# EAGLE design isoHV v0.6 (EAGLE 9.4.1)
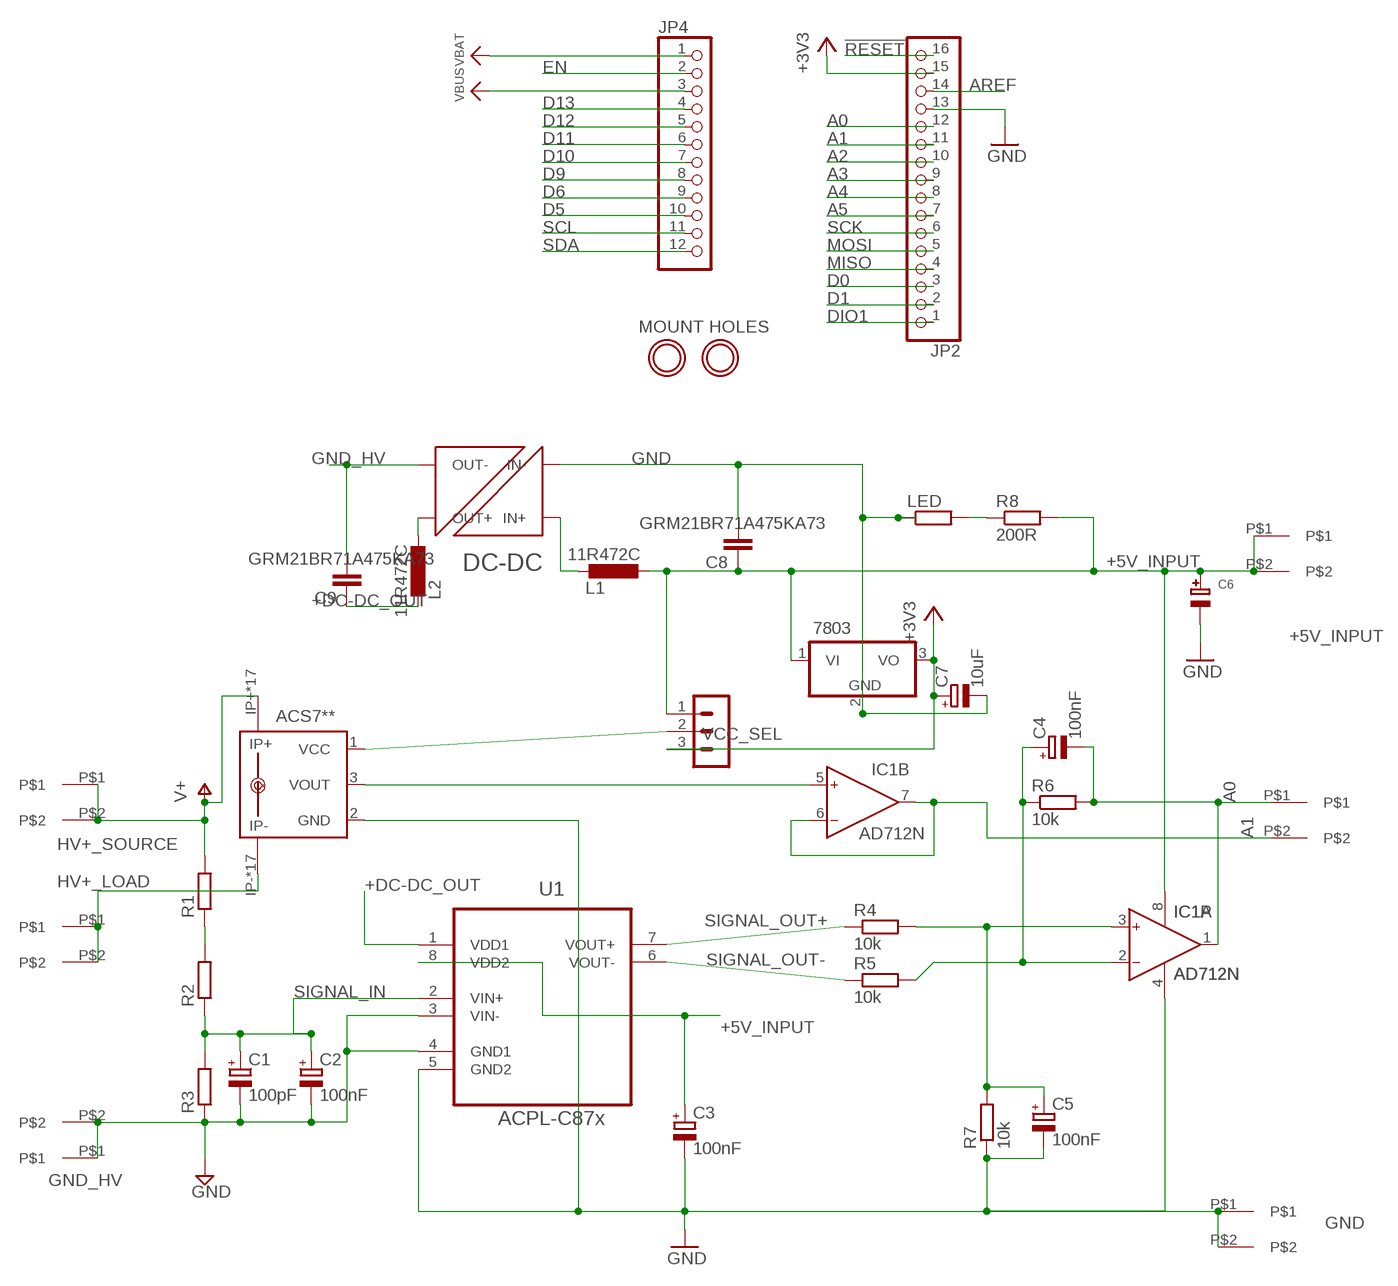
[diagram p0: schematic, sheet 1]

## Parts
7803  7805TV  [TO220V]
ACS7**  ACS758KCB-150B-PFF-T  [CB-PFF]
C1  100pF  CPOL-EUB45181A  [B45181A]
C2  100nF  CPOL-EUB45181A  [B45181A]
C3  100nF  CPOL-EUB45181A  [B45181A]
C4  100nF  CPOL-EUB45181A  [B45181A]
C5  100nF  CPOL-EUB45181A  [B45181A]
C6  CAP_ELECTROLYTICPTH_3.5MMGRID_10MMDIA  [CELEC_3.5MM_10MM]
C7  10uF  CPOL-EUB45181A  [B45181A]
C8  GRM21BR71A475KA73  C-EU025-050X050  [C025-050X050]
C9  GRM21BR71A475KA73  C-EU025-050X050  [C025-050X050]
IC1  AD712N  [DIL08]
JP2  HEADER-1X16ROUND  [1X16_ROUND]
JP4  HEADER-1X12  [1X12_ROUND]
L1  11R472C  L-EU0204V  [0204V]
L2  11R472C  L-EU0204V  [0204V]
LED  R-EU_0204/2V  [0204V]
R1  R-EU_0411/15  [0411/15]
R2  R-EU_0411/15  [0411/15]
R3  R-EU_0411/15  [0411/15]
R4  10k  R-EU_0204/7  [0204/7]
R5  10k  R-EU_0204/7  [0204/7]
R6  10k  R-EU_0204/7  [0204/7]
R7  10k  R-EU_0204/7  [0204/7]
R8  200R  R-EU_0204/2V  [0204V]
U1  ACPL-C87x  ACPL-C79B-000E  [SOIC127P1150X330-8N]
U$1  7.62MM_TERMINAL_BLOCK  [7.62MM]
U$2  7.62MM_TERMINAL_BLOCK  [7.62MM]
U$3  7.62MM_TERMINAL_BLOCK  [7.62MM]
U$4  7.62MM_TERMINAL_BLOCK  [7.62MM]
U$5  7.62MM_TERMINAL_BLOCK  [7.62MM]
U$6  7.62MM_TERMINAL_BLOCK  [7.62MM]
U$7  NXF1  [NXF1]
U$12  MOUNTINGHOLE2.5  [MOUNTINGHOLE_2.5_PLATED]
U$13  MOUNTINGHOLE2.5  [MOUNTINGHOLE_2.5_PLATED]
VCC_SEL  MA03-1  [MA03-1]

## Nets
!RESET: JP2.16
+3V3: 7803.3(VO) C7.+ JP2.15 VCC_SEL.3
+5V_INPUT: 7803.1(VI) C3.+ C6.+ C8.1 IC1.8(P:V+) L1.2 R8.2 U1.8(VDD2) U$3.P$1 U$3.P$2 VCC_SEL.1
+DC-DC_OUT: C9.1 L2.1 U1.1(VDD1)
A0: C4.- IC1.1(A:OUT) JP2.12 R6.2 U$5.P$1
A1: IC1.6(B:IN-) IC1.7(B:OUT) JP2.11 U$5.P$2
A2: JP2.10
A3: JP2.9
A4: JP2.8
A5: JP2.7
AREF: JP2.14
D0: JP2.3
D1: JP2.2
D5: JP4.10
D6: JP4.9
D9: JP4.8
D10: JP4.7
D11: JP4.6
D12: JP4.5
D13: JP4.4
DIO1: JP2.1
EN: JP4.2
GND: 7803.2(GND) ACS7**.2(GND) C3.- C5.- C6.- C7.- C8.2 IC1.4(P:V-) JP2.13 LED.1 R7.1 U1.5(GND2) U$4.P$1 U$4.P$2 U$7.P$1(IN-)
GND_HV: C1.- C2.- C9.2 R3.1 U1.3(VIN-) U1.4(GND1) U$2.P$1 U$2.P$2 U$7.P$7(OUT-) ; supply symbol labelled GND
HV+_LOAD: ACS7**.IP- ACS7**.IP-@2(IP-) ACS7**.IP-@3(IP-) ACS7**.IP-@4(IP-) ACS7**.IP-@5(IP-) ACS7**.IP-@6(IP-) ACS7**.IP-@7(IP-) ACS7**.IP-@8(IP-) ACS7**.IP-@9(IP-) ACS7**.IP-@10(IP-) ACS7**.IP-@11(IP-) ACS7**.IP-@12(IP-) ACS7**.IP-@13(IP-) ACS7**.IP-@14(IP-) ACS7**.IP-@15(IP-) ACS7**.IP-@16(IP-) ACS7**.IP-@17(IP-) U$6.P$1 U$6.P$2
HV+_SOURCE: ACS7**.IP+ ACS7**.IP+@2(IP+) ACS7**.IP+@3(IP+) ACS7**.IP+@4(IP+) ACS7**.IP+@5(IP+) ACS7**.IP+@6(IP+) ACS7**.IP+@7(IP+) ACS7**.IP+@8(IP+) ACS7**.IP+@9(IP+) ACS7**.IP+@10(IP+) ACS7**.IP+@11(IP+) ACS7**.IP+@12(IP+) ACS7**.IP+@13(IP+) ACS7**.IP+@14(IP+) ACS7**.IP+@15(IP+) ACS7**.IP+@16(IP+) ACS7**.IP+@17(IP+) R1.2 U$1.P$1 U$1.P$2 ; supply symbol labelled V+
MISO: JP2.4
MOSI: JP2.5
N$1: C5.+ IC1.3(A:IN+) R4.2 R7.2
N$2: R1.1 R2.2
N$3: ACS7**.1(VCC) VCC_SEL.2
N$4: LED.2 R8.1
N$5: C4.+ IC1.2(A:IN-) R5.2 R6.1
N$6: ACS7**.3(VOUT) IC1.5(B:IN+)
N$7: L1.1 U$7.P$3(IN+)
N$8: L2.2 U$7.P$8(OUT+)
SCK: JP2.6
SCL: JP4.11
SDA: JP4.12
SIGNAL_IN: C1.+ C2.+ R2.1 R3.2 U1.2(VIN+)
SIGNAL_OUT+: R4.1 U1.7(VOUT+)
SIGNAL_OUT-: R5.1 U1.6(VOUT-)
VBAT: JP4.1
VBUS: JP4.3

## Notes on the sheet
- MOUNT HOLES

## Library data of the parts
7803 = linear:78*: Positive VOLTAGE REGULATOR Source: http://cache.national.com/ds/LM/LM78L05.pdf http://www.fairchildsemi.com/ds/LM/LM7805.pdf
ACS7** = allegro:ACS758*: Thermally Enhanced, Fully Integrated, Hall Effect-Based Linear Current Sensor with 100 micro Ohm Current Conductor display layer 49 Reference in BRD and place VIAs on circles Source: http://www.allegromicro.com/en/Products/Part_Numbers/0758/0758.pdf; MPN: ACS7**; OC_FARNELL: 1718995; OC_NEWARK: 04R7129
C1-C5 C7 = rcl:CPOL-EU: POLARIZED CAPACITOR, European symbol; SPICEPREFIX: C
C6 = microbuilder:CAP_ELECTROLYTIC: Electrolytic Capacitors
C8 C9 = rcl:C-EU: CAPACITOR, European symbol; SPICEPREFIX: C
IC1 = analog-devices:AD712: Dual Precision, Low Cost, High Speed BiFET Op Amp Source: http://www.analog.com/static/imported-files/data_sheets/AD712.pdf; MF: ALTERA CORPORATION; MPN: AD712JNZ; OC_FARNELL: 9604898; OC_NEWARK: 59K4554
JP2 = microbuilder:HEADER-1X16: PIN HEADER
JP4 = microbuilder:HEADER-1X12
L1 L2 = rcl:L-EU: INDUCTOR, European symbol; SPICEPREFIX: L
LED R1-R8 = rcl:R-EU_: RESISTOR, European symbol; SPICEPREFIX: R
U1 = Avago_By_element14_Batch_1:ACPL-C79B-000E: Precision Miniature Isolation Amplifiers; DESCRIPTION: Precision Miniature Isolation Amplifiers; MPN: ACPL-C79B-000E; OC_FARNELL: 1854253; OC_NEWARK: 74R5803; PACKAGE: SOIC-8; SUPPLIER: AVAGO TECHNOLOGIES
U$1-U$6 = 7.62mm terminal block:7.62MM_TERMINAL_BLOCK
U$7 = NXF1:NXF1
U$12 U$13 = microbuilder:MOUNTINGHOLE: Mounting Hole
VCC_SEL = con-lstb:MA03-1: PIN HEADER; OC_FARNELL: unknown; OC_NEWARK: unknown

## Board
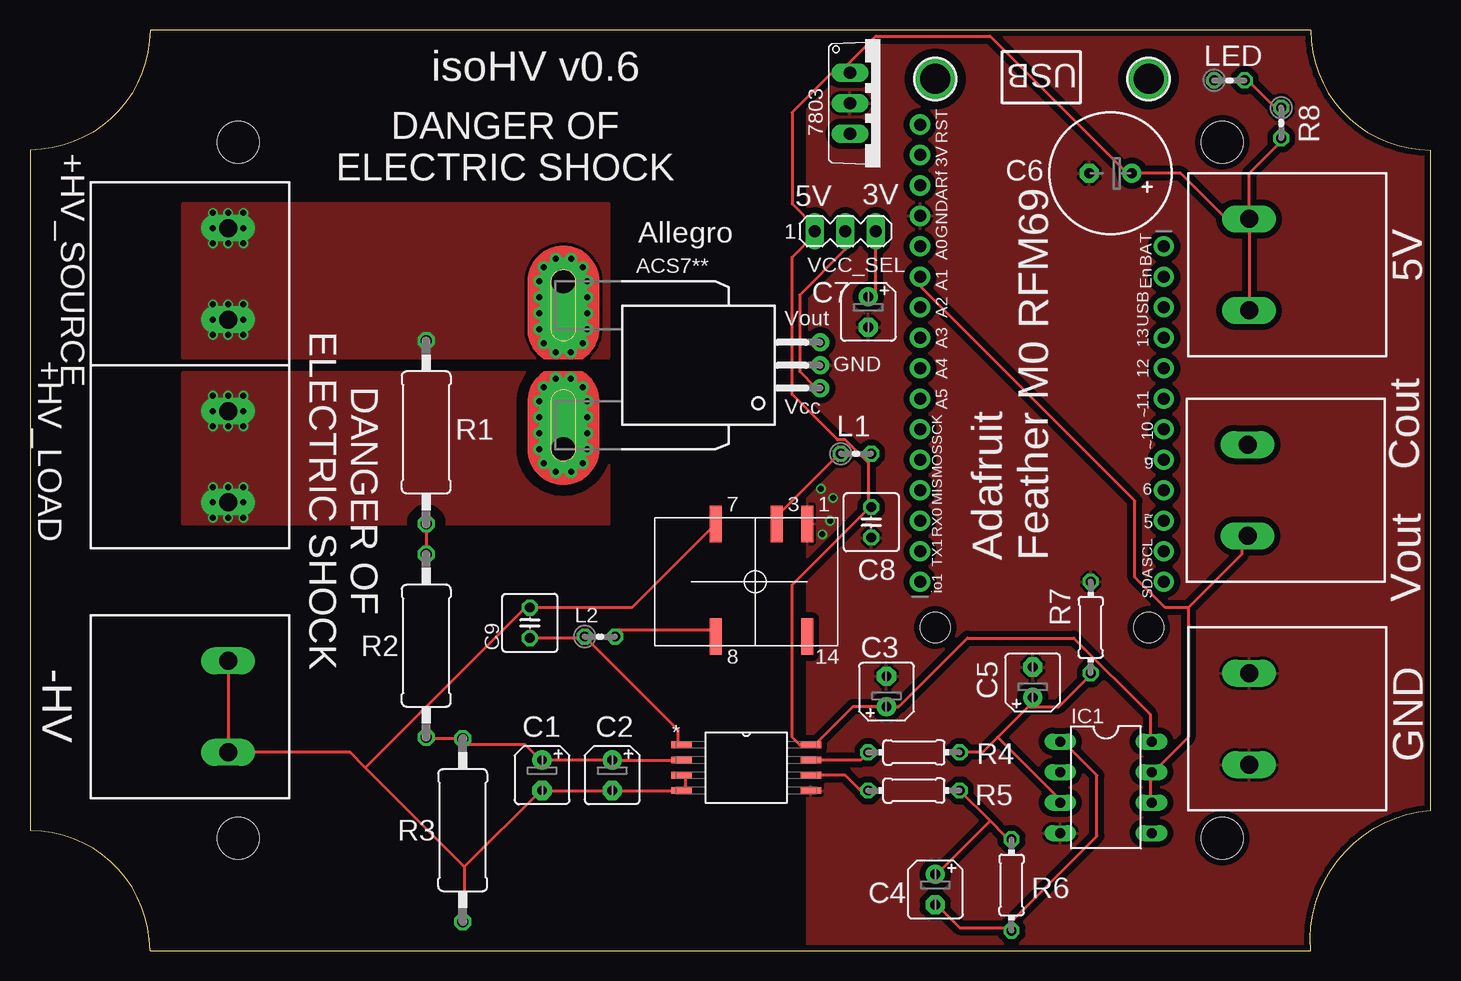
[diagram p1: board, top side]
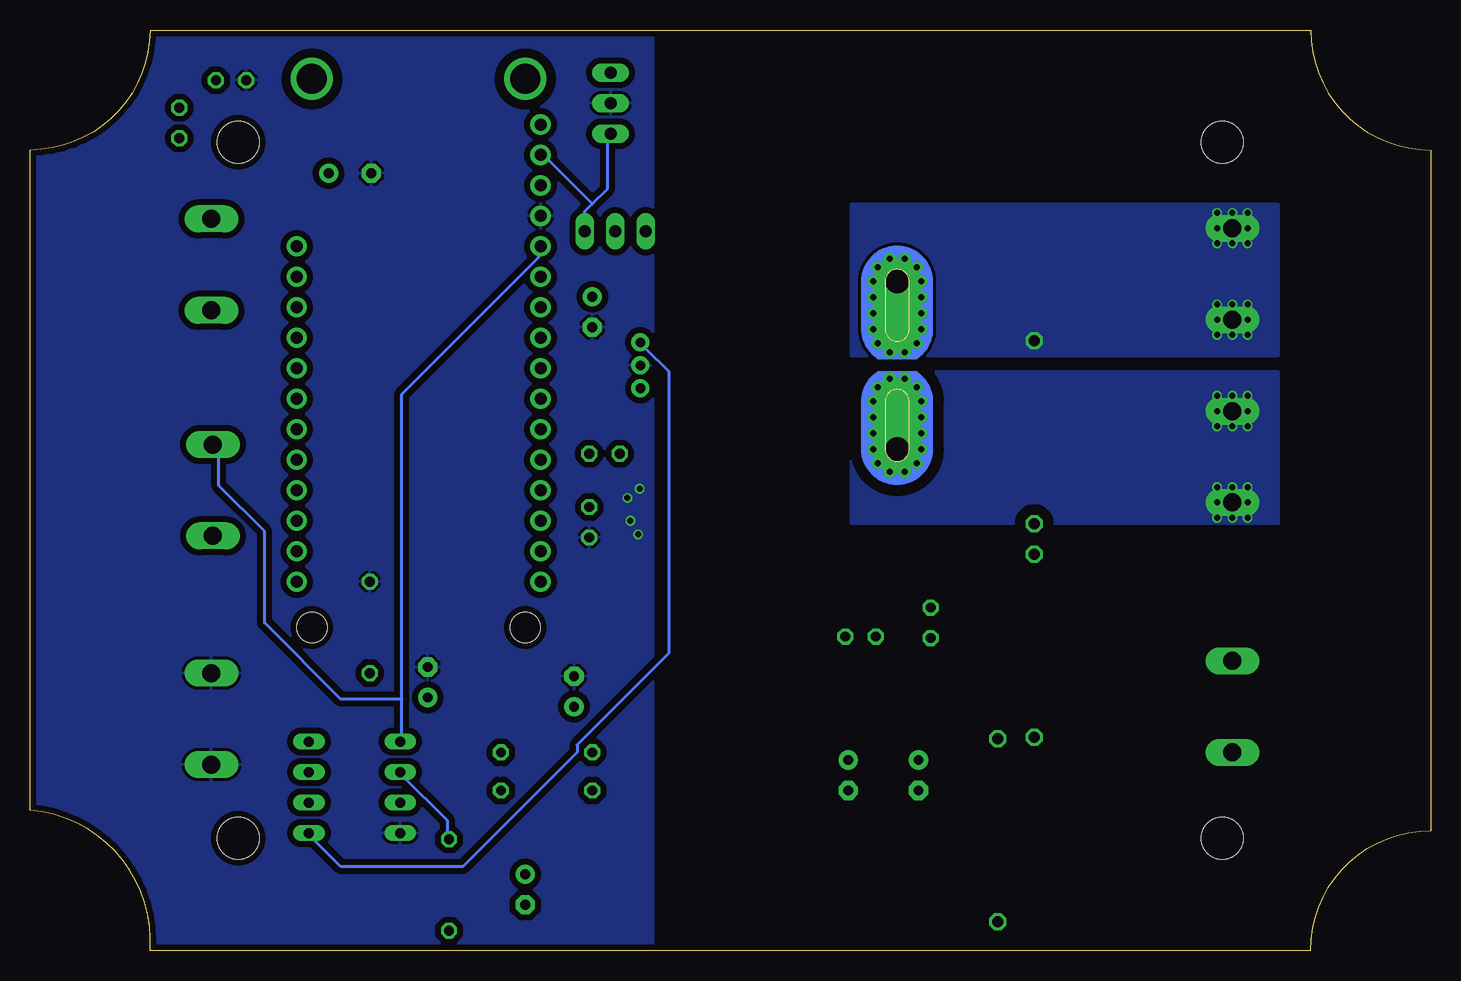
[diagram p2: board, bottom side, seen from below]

Size 116.71 x 76.71 mm. Coordinates in mm from the lower left corner, seen from the top.
Outline: 0,66.71 0,10 arc-90 10,0 106.71,0 arc-90 116.71,11.68 116.71,66.71 arc-90 106.71,76.71 10,76.71 arc-90 0,66.71
Copper layers (1*16): Top 0.07111875mm / dielectric 1.45776875mm / Bottom 0.07111875mm
Design rules "jlcpcb *": minimum track width 10mil, minimum drill 12mil, track to track 10mil, track to pad 10mil, pad to pad 10mil, via to via 10mil, smd to smd 0mil, copper to edge 10mil, drill to drill 10mil, minimum pad ring 10mil, minimum via ring 6mil, stop-mask expansion 2mil, vias tented up to drill 25mil, thermal gap 10mil
Holes 2.5 mm at 93.22,26.92 75.44,26.92
Holes 3.5 mm at 17.36,67.36 99.36,67.36 99.36,9.36 17.36,9.36

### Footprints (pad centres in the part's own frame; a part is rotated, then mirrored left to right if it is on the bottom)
TO220V = drill 1.016 long: 1 -2.54,-2.54; 2 0,-2.54; 3 2.54,-2.54
CB-PFF = drill 0.8 pad 1.5: 1 -1.91,-21.4; 2 0,-21.4; 3 1.91,-21.4 | drill 2 pad 4 offset: IP+ 7,0; IP- -7,0 | drill 0.5 pad 0.9: IP+@2 8.89,0.635; IP+@3 8.89,-0.635; IP+@4 8.175,-1.625; IP+@5 7,-2; IP+@6 5.675,-2; IP+@7 4.35,-2; IP+@8 3,-2; IP+@9 1.825,-1.625; IP+@10 1.1,-0.625; IP+@11 1.1,0.625; IP+@12 1.825,1.625; IP+@13 3,2; IP+@14 4.35,2; IP+@15 5.675,2; IP+@16 7,2; IP+@17 8.175,1.625; IP-@2 -8.89,0.635; IP-@3 -8.89,-0.635; IP-@4 -8.175,-1.625; IP-@5 -7,-2; IP-@6 -5.675,-2; IP-@7 -4.325,-2; IP-@8 -3,-2; IP-@9 -1.825,-1.625; IP-@10 -1.1,-0.625; IP-@11 -1.1,0.625; IP-@12 -1.825,1.625; IP-@13 -3,2; IP-@14 -4.325,2; IP-@15 -5.675,2; IP-@16 -7,2; IP-@17 -8.175,1.625
B45181A = drill 0.813 pad 1.6: + -1.27,0 | drill 0.813 pad 1.6 octagon: - 1.27,0
CELEC_3.5MM_10MM = drill 0.813 pad 1.6: + -1.778,0 | drill 0.813 pad 1.6 octagon: - 1.778,0
C025-050X050 = drill 0.813 octagon: 1 -1.27,0; 2 1.27,0
DIL08 = drill 0.813 long: 1 -3.81,-3.81; 2 -1.27,-3.81; 3 1.27,-3.81; 4 3.81,-3.81; 5 3.81,3.81; 6 1.27,3.81; 7 -1.27,3.81; 8 -3.81,3.81
1X16_ROUND = drill 1 pad 1.676: 1 -19.05,0; 2 -16.51,0; 3 -13.97,0; 4 -11.43,0; 5 -8.89,0; 6 -6.35,0; 7 -3.81,0; 8 -1.27,0; 9 1.27,0; 10 3.81,0; 11 6.35,0; 12 8.89,0; 13 11.43,0; 14 13.97,0; 15 16.51,0; 16 19.05,0
1X12_ROUND = drill 1 pad 1.676: 1 -13.97,0; 2 -11.43,0; 3 -8.89,0; 4 -6.35,0; 5 -3.81,0; 6 -1.27,0; 7 1.27,0; 8 3.81,0; 9 6.35,0; 10 8.89,0; 11 11.43,0; 12 13.97,0
0204V = drill 0.813 octagon: 1 -1.27,0; 2 1.27,0
0411/15 = drill 0.914 octagon: 1 -7.62,0; 2 7.62,0
0204/7 = drill 0.813 octagon: 1 -3.81,0; 2 3.81,0
SOIC127P1150X330-8N = smd 1.702 x 0.559: 1 -5.385,1.905; 2 -5.385,0.635; 3 -5.385,-0.635; 4 -5.385,-1.905; 5 5.385,-1.905; 6 5.385,-0.635; 7 5.385,0.635; 8 5.385,1.905
7.62MM = drill 1.5 long: P$1 0,-3.81; P$2 0,3.81
NXF1 = smd 0.991 x 3.048: P$1 0,0; P$3 2.54,0; P$7 7.62,0; P$8 7.62,9.398; P$14 0,9.398
MOUNTINGHOLE_2.5_PLATED = drill 2.5 pad 3.2: P$1 0,0
MA03-1 = drill 1.016 long: 1 -2.54,0; 2 0,0; 3 2.54,0

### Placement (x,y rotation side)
7803  70.87,70.61 270 top
ACS7**  44.45,48.77 90 top
C1  42.67,14.61 270 top
C2  48.51,14.61 270 top
C3  71.37,21.59 90 top
C4  75.44,5.08 270 top
C5  83.57,22.35 90 top
C6  90.04,64.77 180 top
C7  69.85,53.21 270 top
C8  70.1,35.69 270 top
C9  41.66,27.3 90 top
IC1  89.66,13.59 270 top
JP2  74.17,49.78 90 top
JP4  94.49,44.7 270 top
L1  68.83,41.4 0 top
L2  47.5,26.16 0 top
LED  99.95,72.52 0 top
R1  33.02,43.18 90 top
R2  33.02,25.4 90 top
R3  36.07,10.03 90 top
R4  73.66,16.51 0 top
R5  73.66,13.34 0 top
R6  81.79,5.46 270 top
R7  88.39,26.92 270 top
R8  104.27,68.96 270 top
U1  59.69,15.24 0 top
U$1  16.51,56.39 0 top
U$2  16.51,20.32 0 top
U$3  101.6,57.15 180 top
U$4  101.6,19.3 180 top
U$5  101.47,38.35 180 top
U$6  16.51,41.15 0 top
U$7  64.77,35.56 180 top
U$12  93.22,72.64 270 top
U$13  75.44,72.64 270 top
VCC_SEL  67.94,59.94 0 top

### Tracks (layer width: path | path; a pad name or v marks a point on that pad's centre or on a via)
+3V3
  Top 0.254: VCC_SEL.3 70.48,54.61 69.85,53.98 C7.+
  Bottom 0.254: 69.85,62.23 70.48,61.59 VCC_SEL.3 | 69.85,62.23 68.58,63.5 68.58,67.94 7803.3 | 69.85,62.23 73.66,66.04 JP2.15
+5V_INPUT
  Top 0.254: U$3.P$1 101.6,64.77 104.14,67.31 R8.2 | U$3.P$1 99.69,60.96 95.89,64.77 C6.+ 91.44,64.77 80.01,76.2 70.48,76.2 67.94,73.66 7803.1 67.94,73.03 66.67,73.03 63.5,69.85 63.5,62.23 65.41,60.33 VCC_SEL.1 65.41,59.69 63.5,57.78 63.5,46.35 67.31,42.55 67.94,42.55 69.85,40.64 | U$3.P$1 U$3.P$2 | 69.85,40.64 69.85,41.27 L1.2 | 69.85,40.64 69.85,37.47 C8.1 69.85,36.83 63.5,30.48 63.5,17.78 64.14,17.14 U1.8 65.41,17.14 68.58,20.32 C3.+ 72.39,20.32 78.11,26.04 87,26.04 93.34,19.68 93.34,17.78 IC1.8
+DC-DC_OUT
  Top 0.254: U1.1 53.98,17.14 53.98,18.41 L2.1 45.72,26.04 C9.1
A0
  Top 0.254: 81.28,1.91 77.47,1.91 75.56,3.81 C4.- | 81.28,1.91 88.9,9.53 88.9,14.61 86.36,17.14 IC1.1 | 81.28,1.91 R6.2
  Bottom 0.254: 85.72,20.95 85.72,17.78 IC1.1 | 85.72,20.95 85.72,46.35 74.3,57.78 74.3,58.42 JP2.12 | 85.72,20.95 90.81,20.95 97.16,27.3 97.16,34.92 100.97,38.73 100.97,41.91 U$5.P$1
A1
  Top 0.254: IC1.6 93.34,12.7 93.34,14.61 IC1.7 93.98,15.24 96.52,17.78 96.52,28.57 | 96.52,28.57 94.61,28.57 92.08,31.11 92.08,37.47 74.3,55.24 74.3,55.88 JP2.11 | 96.52,28.57 100.97,33.02 100.97,34.29 U$5.P$2
GND  (via drill 0.5)
  other vias: 65.91,38.48 66.93,37.72 66.67,35.81 66.04,34.67
  pour Bottom (isolate 0.508): 64.77,77.47 118.11,77.47 118.11,-1.27 64.77,-1.27
  pour Top (isolate 0.508): 64.77,78.74 64.77,-2.54 119.38,-2.54 119.38,78.74
GND_HV
  Top 0.254: U$7.P$7 50.16,28.57 C9.2 41.27,28.57 27.94,15.24 | U$2.P$2 U$2.P$1 26.67,16.51 27.94,15.24 | U1.3 54.61,14.61 54.61,13.34 U1.4 C2.- C1.- 42.55,13.34 36.2,6.99 | 36.2,6.99 36.2,2.54 R3.1 | 36.2,6.99 27.94,15.24
HV+_LOAD  (via drill 0.5)
  other vias: 16.51,43.69 15.24,46.23 16.51,46.23 17.78,46.23 17.78,44.96 17.78,43.69 15.24,43.69 15.24,44.96 17.78,38.61 17.78,37.34 17.78,36.07 16.51,36.07 15.24,36.07 15.24,37.34 15.24,38.61 16.51,38.61
  pour Bottom (isolate 0.889, no thermals): 48.26,48.26 12.7,48.26 12.7,35.56 48.26,35.56
  pour Top (isolate 0.889, no thermals): 48.26,48.13 12.7,48.13 12.7,35.56 48.26,35.56
HV+_SOURCE  (via drill 0.5)
  other vias: 15.24,53.85 16.51,53.85 17.78,53.85 17.78,52.58 17.78,51.31 16.51,51.31 15.24,51.31 15.24,52.58 16.51,58.93 17.78,58.93 17.78,60.2 17.78,61.47 16.51,61.47 15.24,61.47 15.24,60.2 15.24,58.93
  pour Bottom (no thermals): 12.7,49.53 48.26,49.53 48.26,62.23 12.7,62.23
  pour Top (no thermals): 12.7,49.4 48.26,49.4 48.26,62.23 12.7,62.23
N$1
  Top 0.254: R4.2 79.38,16.51 80.64,17.78 | 83.19,20.32 83.82,20.95 C5.+ | 83.19,20.32 80.64,17.78 | 80.64,17.78 85.72,12.7 IC1.3 | 83.19,20.32 85.72,20.32 88.27,22.86 R7.2
N$2
  Top 0.254: R1.1 R2.2
N$3
  Top 0.254: VCC_SEL.2 67.94,58.42 64.14,54.61 64.14,48.26 65.41,46.99 ACS7**.1
N$4
  Top 0.254: LED.2 101.6,72.39 104.14,69.85 R8.1
N$5
  Top 0.254: 80.01,10.79 81.28,9.53 R6.1 | 80.01,10.79 R5.2 | 80.01,10.79 75.56,6.35 C4.+
  Bottom 0.254: IC1.2 85.72,14.61 81.92,10.79 81.92,9.53 R6.1
N$6
  Bottom 0.254: IC1.5 93.34,9.53 90.81,6.99 80.64,6.99 71.12,16.51 71.12,17.14 63.5,24.77 63.5,48.26 65.41,50.16 ACS7**.3
N$7
  Top 0.254: U$7.P$3 62.23,36.2 67.31,41.27 L1.1
N$8
  Top 0.254: L2.2 48.9,26.67 57.15,26.67 U$7.P$8
SIGNAL_IN
  Top 0.254: R2.1 33.15,17.65 R3.2 36.2,17.14 41.27,17.14 42.55,15.88 C1.+ C2.+ U1.2
SIGNAL_OUT+
  Top 0.254: U1.7 69.22,15.88 R4.1
SIGNAL_OUT-
  Top 0.254: U1.6 67.94,14.61 69.22,13.34 R5.1

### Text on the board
tPlace: USB | RST | 3V | ARf | GND | A0 | BAT | A1 | En | A2 | USB | A3 | 13 | A4 | 12 | A5 | 11 | ~ | SCK | 10 | ~ | MOS | 9 | ~ | MIS | 6 | RX0 | 5 | ~ | TX1 | Adafruit / Feather M0 RFM69 | SCL | io1 | SDA
tNames: isoHV v0.6 | DANGER OF / ELECTRIC SHOCK | +HV_SOURCE | 5V | 3V | Allegro | 5V | Vout | +HV_LOAD | GND | Vcc | Cout | DANGER OF / ELECTRIC SHOCK | Vout | -HV | GND

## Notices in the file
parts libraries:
microbuilder: This work is placed in the public domain, and may be freely used for commercial and non-commercial work with the following conditions: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
